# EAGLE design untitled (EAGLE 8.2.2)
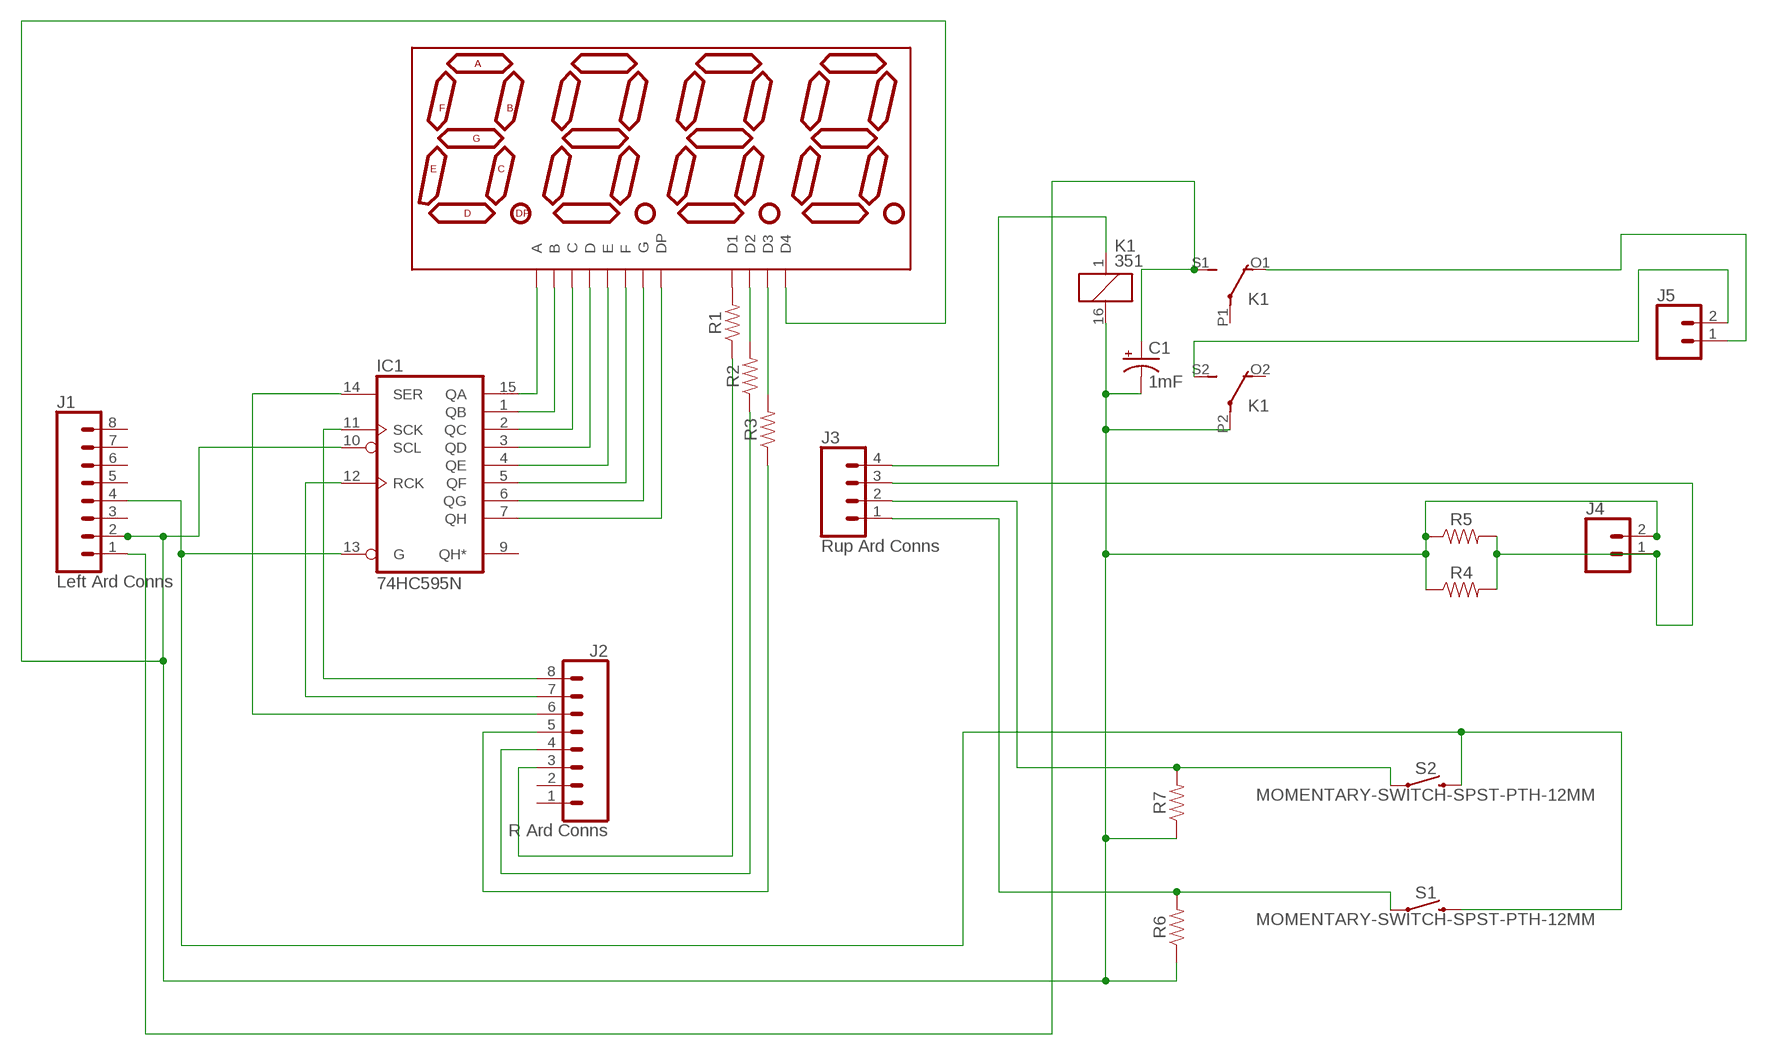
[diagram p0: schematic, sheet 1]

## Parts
C1  1mF  1000UF-RADIAL-5MM-25V-20%  [CPOL-RADIAL-5MM-10MM]
DISP1  7-SEGMENT-4DIGIT-20MM-HP-BUBBLE  [DIP12-HP-BUBBLE]
IC1  74HC595N  [DIL16]
J1  Left Ard Conns  CONN_08"  [1X08]
J2  R Ard Conns  CONN_08"  [1X08]
J3  Rup Ard Conns  CONN_04  [1X04]
J4  CONN_025MM  [SCREWTERMINAL-5MM-2]
J5  CONN_025MM  [SCREWTERMINAL-5MM-2]
K1  351  [351]
R1  RESISTORAXIAL-0.3  [AXIAL-0.3]
R2  RESISTORAXIAL-0.3  [AXIAL-0.3]
R3  RESISTORAXIAL-0.3  [AXIAL-0.3]
R4  RESISTORAXIAL-0.3  [AXIAL-0.3]
R5  RESISTORAXIAL-0.3  [AXIAL-0.3]
R6  RESISTORAXIAL-0.3  [AXIAL-0.3]
R7  RESISTORAXIAL-0.3  [AXIAL-0.3]
S1  MOMENTARY-SWITCH-SPST-PTH-12MM  [TACTILE_SWITCH_PTH_12MM]
S2  MOMENTARY-SWITCH-SPST-PTH-12MM  [TACTILE_SWITCH_PTH_12MM]

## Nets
N$1: DISP1.12(A) IC1.15(QA)
N$2: DISP1.11(B) IC1.1(QB)
N$3: DISP1.3(C) IC1.2(QC)
N$4: DISP1.8(D) IC1.3(QD)
N$5: DISP1.2(E) IC1.4(QE)
N$6: DISP1.9(F) IC1.5(QF)
N$7: DISP1.7(G) IC1.6(QG)
N$8: DISP1.5(DP) IC1.7(QH)
N$9: DISP1.1(D1) R1.P$2
N$10: DISP1.10(D2) R2.P$2
N$11: DISP1.4(D3) R3.P$2
N$12: J2.3 R1.P$1
N$13: J2.4 R2.P$1
N$14: J2.5 R3.P$1
N$15: IC1.12(RCK) J2.7
N$16: IC1.13(G) J1.4 S1.3 S2.3
N$17: IC1.14(SER) J2.6
N$18: IC1.11(SCK) J2.8
N$19: C1.- DISP1.6(D4) IC1.10(SCL) J1.2 J4.2 K1.16 K1.P2(3:P) R4.P$1 R5.P$1 R6.P$1 R7.P$1
N$20: J3.1 R6.P$2 S1.1
N$21: J3.2 R7.P$2 S2.1
N$22: J3.3 J4.1 R4.P$2 R5.P$2
N$25: J3.4 K1.1
N$26: J5.2 K1.S2(3:S)
N$27: J5.1 K1.O1(2:O)
N$28: C1.+ J1.1 K1.S1(2:S)
Unconnected: IC1.9(QH*) J1.3 J1.5 J1.6 J1.7 J1.8 J2.1 J2.2 K1.O2(3:O) K1.P1(2:P)

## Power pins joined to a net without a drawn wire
GND: IC1.8(GND)
VCC: IC1.16(VCC)

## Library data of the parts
C1 = SparkFun-Capacitors:1000UF: 1,000µF/1mF ceramic capacitors; PROD_ID: CAP-09538
DISP1 = SparkFun-LED:7-SEGMENT-4DIGIT-20MM: 4 Digit 7 Segment Display This is a part for the 4-Digit 7-segment LEDs from Young Sun. Different from the Digikey LEDs, all 16 pins are used. The LONGPADS Variant is used for a test jig, but you may like it because there is more pad to solder to. If you are concerned about routing space, the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; STOREFRONT: COM-12710
IC1 = 74xx-eu:74*595: 8-bit SHIFT REGISTER, output latch
J1 J2 = SparkFun-Connectors:CONN_08: Multi connection point. Often used as Generic Header-pin footprint for 0.1 inch spaced/style header connections On any of the 0.1 inch spaced packages, you can populate with these: Break Away Headers - Straight (PRT-00116) Break Away Male Headers - Right Angle (PRT-00553) Female Headers (PRT-00115)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; PROD_ID: CONN-08438
J3 = SparkFun-Connectors:CONN_04: Multi connection point. Often used as Generic Header-pin footprint for 0.1 inch spaced/style header connections On any of the 0.1 inch spaced packages, you can populate with these: Break Away Headers - Straight (PRT-00116) Break Away Male Headers - Right Angle (PRT-00553) Female Headers (PRT-00115)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; PROD_ID: CONN-09696
J4 J5 = SparkFun-Connectors:CONN_02: Multi connection point. Often used as Generic Header-pin footprint for 0.1 inch spaced/style header connections; SF_SKU: PRT-08432
K1 = relay:351: RELAY 2 x switch, Omron; OC_FARNELL: unknown; OC_NEWARK: unknown
R1-R7 = SparkFun-Resistors:RESISTOR: Generic Resistor Package
S1 S2 = SparkFun-Switches:MOMENTARY-SWITCH-SPST: Momentary Switch (Pushbutton) - SPST; PROD_ID: SWCH-09185; SF_SKU: COM-09190

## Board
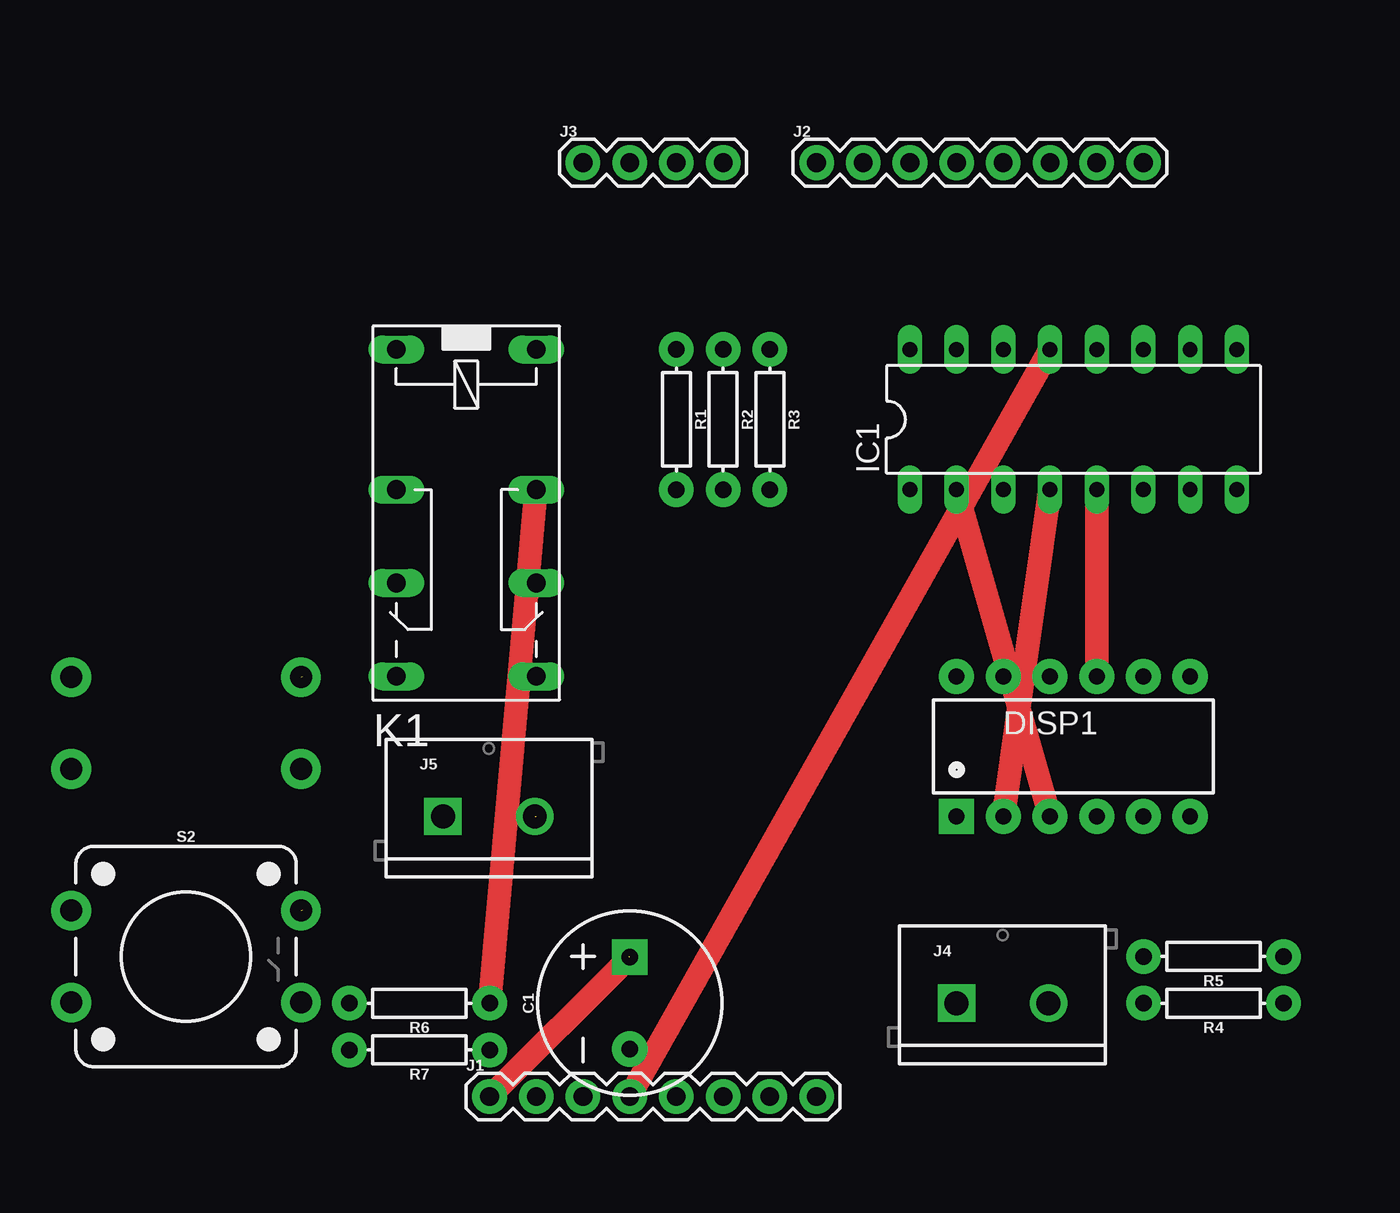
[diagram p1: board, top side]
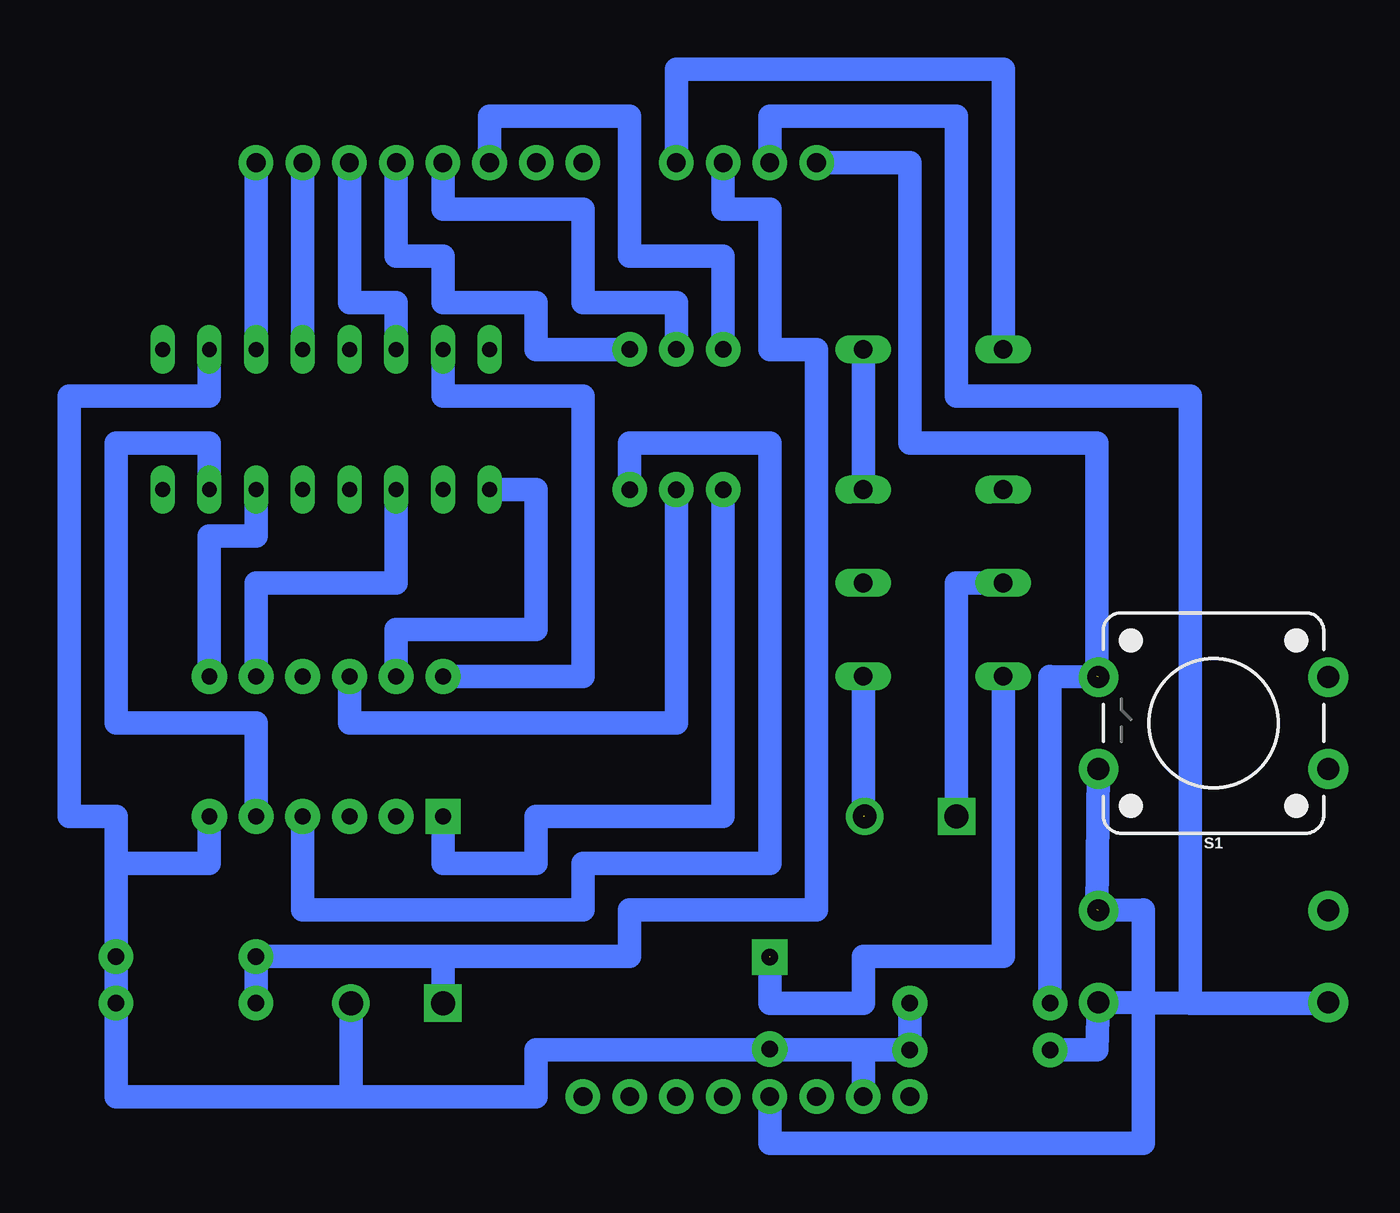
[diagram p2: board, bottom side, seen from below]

No outline drawn. Coordinates in mm, seen from the top.
Copper layers 1+16: Top 0.035mm / dielectric 1.5mm / Bottom 0.035mm
Design rules "default *": minimum track width 50mil, minimum drill 0.35mm, track to track 50mil, track to pad 50mil, pad to pad 6mil, via to via 6mil, smd to smd 6mil, copper to edge 40mil, drill to drill 6mil, minimum pad ring 10mil, minimum via ring 8mil, stop-mask expansion 4mil, vias tented up to drill 0mil, thermal gap 10mil

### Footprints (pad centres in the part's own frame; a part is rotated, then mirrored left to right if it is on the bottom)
CPOL-RADIAL-5MM-10MM = drill 0.9 pad 1.93 square: + 2.5,0 | drill 0.9 pad 1.93: - -2.5,0
DIP12-HP-BUBBLE = drill 0.864 pad 1.905 square: 1 -6.35,-3.81 | drill 0.864 pad 1.905: 2 -3.81,-3.81; 3 -1.27,-3.81; 4 1.27,-3.81; 5 3.81,-3.81; 6 6.35,-3.81; 7 6.35,3.81; 8 3.81,3.81; 9 1.27,3.81; 10 -1.27,3.81; 11 -3.81,3.81; 12 -6.35,3.81
DIL16 = drill 0.813 long: 1 -8.89,-3.81; 2 -6.35,-3.81; 3 -3.81,-3.81; 4 -1.27,-3.81; 5 1.27,-3.81; 6 3.81,-3.81; 7 6.35,-3.81; 8 8.89,-3.81; 9 8.89,3.81; 10 6.35,3.81; 11 3.81,3.81; 12 1.27,3.81; 13 -1.27,3.81; 14 -3.81,3.81; 15 -6.35,3.81; 16 -8.89,3.81
1X08 = drill 1.016 pad 1.88: 1 0,0; 2 2.54,0; 3 5.08,0; 4 7.62,0; 5 10.16,0; 6 12.7,0; 7 15.24,0; 8 17.78,0
1X04 = drill 1.016 pad 1.88: 1 0,0; 2 2.54,0; 3 5.08,0; 4 7.62,0
SCREWTERMINAL-5MM-2 = drill 1.3 pad 2.032 square: 1 0,0 | drill 1.3 pad 2.032: 2 5,0
351 = drill 1.016 long: 1 -3.81,-3.81; 16 -3.81,3.81; O1 8.89,-3.81; O2 8.89,3.81; P1 3.81,-3.81; P2 3.81,3.81; S1 13.97,-3.81; S2 13.97,3.81
AXIAL-0.3 = drill 0.9 pad 1.88: P$1 -3.81,0; P$2 3.81,0
TACTILE_SWITCH_PTH_12MM = drill 1.2 pad 2.159: 1 6.25,-2.5; 2 -6.25,-2.5; 3 6.25,2.5; 4 -6.25,2.5

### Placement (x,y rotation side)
C1  60.96,25.4 90 top
DISP1  85.09,39.37 0 top
IC1  85.09,57.15 0 top
J1  53.34,20.32 0 top
J2  71.12,71.12 0 top
J3  58.42,71.12 0 top
J4  78.74,25.4 0 top
J5  50.8,35.56 0 top
K1  52.07,57.15 270 top
R1  63.5,57.15 270 top
R2  66.04,57.15 270 top
R3  68.58,57.15 270 top
R4  92.71,25.4 180 top
R5  92.71,27.94 180 top
R6  49.53,25.4 180 top
R7  49.53,22.86 180 top
S1  36.83,40.64 180 bottom
S2  36.83,27.94 0 top

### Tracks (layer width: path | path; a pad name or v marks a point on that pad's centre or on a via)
N$1
  Bottom 1.27: DISP1.12 71.12,43.18 71.12,58.42 78.74,58.42 IC1.15
N$2
  Bottom 1.27: DISP1.11 81.28,45.72 73.66,45.72 73.66,53.34 IC1.1
N$3
  Top 1.27: IC1.2 DISP1.3
N$4
  Bottom 1.27: DISP1.8 88.9,48.26 81.28,48.26 IC1.3
N$5
  Top 1.27: IC1.4 DISP1.2
N$6
  Top 1.27: IC1.5 DISP1.9
N$7
  Bottom 1.27: DISP1.7 91.44,50.8 88.9,50.8 IC1.6
N$8
  Bottom 1.27: DISP1.5 88.9,40.64 96.52,40.64 96.52,55.88 91.44,55.88 IC1.7
N$9
  Bottom 1.27: R1.P$2 63.5,35.56 73.66,35.56 73.66,33.02 78.74,33.02 DISP1.1
N$10
  Bottom 1.27: R2.P$2 66.04,40.64 83.82,40.64 DISP1.10
N$11
  Bottom 1.27: R3.P$2 68.58,55.88 60.96,55.88 60.96,33.02 71.12,33.02 71.12,30.48 86.36,30.48 DISP1.4
N$12
  Bottom 1.27: R1.P$1 63.5,66.04 68.58,66.04 68.58,73.66 76.2,73.66 J2.3
N$13
  Bottom 1.27: R2.P$1 66.04,63.5 71.12,63.5 71.12,68.58 78.74,68.58 J2.4
N$14
  Bottom 1.27: R3.P$1 73.66,60.96 73.66,63.5 78.74,63.5 78.74,66.04 81.28,66.04 J2.5
N$15
  Bottom 1.27: IC1.12 J2.7
N$16  (1 unrouted)
  Top 1.27: IC1.13 J1.4
  Bottom 1.27: S1.3 43.18,30.48 | S2.3 40.64,30.48 40.64,17.78 60.96,17.78 J1.4
N$17
  Bottom 1.27: IC1.14 81.28,63.5 83.82,63.5 J2.6
N$18
  Bottom 1.27: IC1.11 J2.8
N$19
  Top 1.27: K1.P2 R6.P$1
  Bottom 1.27: 96.52,33.02 R5.P$1 R4.P$1 96.52,20.32 83.82,20.32 | 96.52,33.02 96.52,35.56 99.06,35.56 99.06,58.42 91.44,58.42 IC1.10 | R6.P$1 R7.P$1 55.88,22.86 | 55.88,22.86 68.58,22.86 | 68.58,22.86 C1.- | K1.16 K1.P2 | J1.2 55.88,22.86 | 68.58,22.86 73.66,22.86 73.66,20.32 83.82,20.32 | J4.2 83.74,20.4 83.82,20.32 | 96.52,33.02 91.44,33.02 DISP1.6
N$20  (1 unrouted)
  Bottom 1.27: S1.1 45.72,43.18 R6.P$2 | J3.1 53.34,71.12 53.34,55.88 43.18,55.88 43.18,43.18
N$21
  Bottom 1.27: R7.P$2 43.18,22.86 S2.1 38.1,25.4 | 38.1,25.4 38.1,58.42 50.8,58.42 50.8,73.66 60.96,73.66 J3.2 | 38.1,25.4 30.48,25.4
N$22
  Bottom 1.27: R4.P$2 R5.P$2 79.38,27.94 | J3.3 63.5,68.58 60.96,68.58 60.96,60.96 58.42,60.96 58.42,30.48 68.58,30.48 68.58,27.94 79.38,27.94 | J4.1 78.74,27.94 79.38,27.94
N$25
  Bottom 1.27: K1.1 48.26,76.2 66.04,76.2 J3.4
N$26  (1 unrouted)
  Bottom 1.27: K1.S2 55.88,35.56
N$27
  Bottom 1.27: K1.O1 50.8,48.26 J5.1
N$28  (1 unrouted)
  Top 1.27: C1.+ J1.1
  Bottom 1.27: K1.S1 48.26,27.94 55.88,27.94 55.88,25.4 60.96,25.4 60.96,27.94

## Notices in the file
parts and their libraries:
SparkFun-Resistors: Licensing: Creative Commons ShareAlike 4.0 International - https://creativecommons.org/licenses/by-sa/4.0
